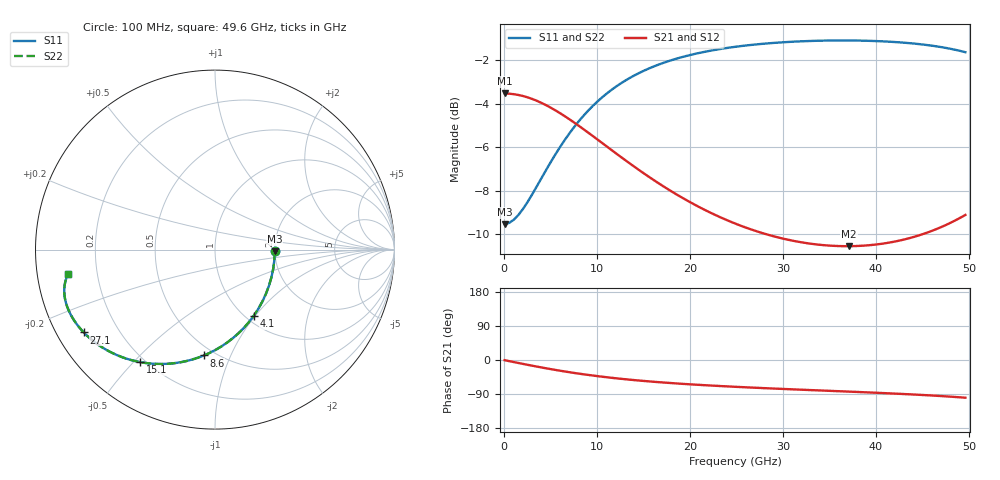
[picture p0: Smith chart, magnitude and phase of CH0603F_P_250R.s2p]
# GHz S RI R 250
! S-Parameters data
! Freq  reS11  imS11  reS21  imS21  reS12  imS12  reS22  imS22
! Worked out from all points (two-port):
!   100 points, 100 MHz to 49.6 GHz, reference 250 ohm
!   highest |S21| = -3.52 dB at 100 MHz (marker M1); lowest = -10.6 dB at 37.1 GHz (marker M2)
!   |S21| within 3 dB of the highest: start of sweep to 12.84 GHz
!   lowest |S11| = -9.5 dB at 100 MHz (marker M3), VSWR 2.00, Z = 500 - j11.1 ohm
!   |S11| at or under -10 dB: nowhere
!   |S22| runs from -9.5 to -1.1 dB; largest |S21 - S12| = 0
!   S11 on the Smith chart (normalised r, x): 100 MHz: 2.00, -0.04; 4.1 GHz: 1.09, -0.98; 8.6 GHz: 0.44, -0.80; 15.1 GHz: 0.18, -0.52; 27.1 GHz: 0.08, -0.29; 49.6 GHz: 0.09, -0.08
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0.1  0.3333 -0.00988  0.6666 -0.00582  0.6666 -0.00582  0.3333 -0.00988
1.1  0.3241 -0.1079  0.6611 -0.0636  0.6611 -0.0636  0.3241 -0.1079
2.1  0.3004 -0.2022  0.6466 -0.1189  0.6466 -0.1189  0.3004 -0.2022
4.1  0.2161 -0.3684  0.596 -0.2151  0.596 -0.2151  0.2161 -0.3684
5.1  0.1605 -0.4366  0.563 -0.2537  0.563 -0.2537  0.1605 -0.4366
6.1  0.0993 -0.4937  0.5273 -0.2856  0.5273 -0.2856  0.0993 -0.4937
7.1  0.0352 -0.5398  0.4904 -0.3109  0.4904 -0.3109  0.0352 -0.5398
8.6  -0.0622 -0.5899  0.4356 -0.3377  0.4356 -0.3377  -0.0622 -0.5899
10.1  -0.1563 -0.6202  0.3839 -0.3535  0.3839 -0.3535  -0.1563 -0.6202
11.6  -0.244 -0.6347  0.3369 -0.361  0.3369 -0.361  -0.244 -0.6347
13.1  -0.3236 -0.6371  0.2952 -0.3625  0.2952 -0.3625  -0.3236 -0.6371
15.1  -0.4166 -0.627  0.2477 -0.3587  0.2477 -0.3587  -0.4166 -0.627
16.6  -0.4768 -0.6126  0.2176 -0.3532  0.2176 -0.3532  -0.4768 -0.6126
18.6  -0.5455 -0.5881  0.1837 -0.3442  0.1837 -0.3442  -0.5455 -0.5881
20.6  -0.6028 -0.5599  0.1557 -0.3346  0.1557 -0.3346  -0.6028 -0.5599
25.1  -0.6992 -0.492  0.1085 -0.3149  0.1085 -0.3149  -0.6992 -0.492
27.1  -0.7308 -0.4618  0.0925 -0.308  0.0925 -0.308  -0.7308 -0.4618
33.1  -0.797 -0.3747  0.0548 -0.2954  0.0548 -0.2954  -0.797 -0.3747
37.1  -0.8231 -0.3192  0.0338 -0.2948  0.0338 -0.2948  -0.8231 -0.3192
41.6  -0.8382 -0.2569  0.00952 -0.3028  0.00952 -0.3028  -0.8382 -0.2569
46.1  -0.8366 -0.1915  -0.0217 -0.3217  -0.0217 -0.3217  -0.8366 -0.1915
49.6  -0.8183 -0.1362  -0.0581 -0.3454  -0.0581 -0.3454  -0.8183 -0.1362
